| TEXAS INSTRUMENTS INCORPORATED
| Standard Linear and Logic Group
| IBIS Model of SN74LVC16646A
| 16-BIT REGISTERED TRANCEIVER AND REGISTER WITH 3-STATE OUTPUTS
| This file contains package information for the following:
|  TSSOP 56-pin (DGG) package as [Component] LVC16646A_DGG
|  TVSOP 56-pin (DGV) package as [Component] LVC16646A_DGV
|  SSOP 56-pin (DL) package as [Component] LVC16646A_DL
| This device can be powered at the following Vccs:
|  1.8 volt Vcc
|  2.5 volt Vcc
|  3.3 volt Vcc
| This file provides unique models under the [Model Selector] for each Vcc.
| For operation at a specific Vcc, select the appropriate model after each
| [Model Selector] keyword.
[IBIS Ver]   3.2
[Comment char]  |_char
[File Name]   sn74lvc16646a.ibs
[File Rev]   1.1 | c_die
[Date]   September 3, 2002
[Source]   Data created from TI-SPICE simulations at TI-SLL.
[Notes]   The following is an IBIS list for the LVC16646A.
   Please contact sllibis@ti.com with questions and
   comments concerning SLL IBIS models.
   This IBIS model is created from a BA (back annotated netlist
   - Power-clamp data has been deleted since there is no
   power-clamp diode in the device.
   - Due to the fact that the device is 5-V input/output
   tolerant, the pullup data has some non-monotonic warnings.
   - End point warning due to AC and DC mismatch.
[Disclaimer] Property of Texas Instruments Incorporated.  Unauthorized
   reproduction and/or distribution is strictly prohibited.
   This product is protected under copyright law.
   Created  2002, (C) Copyright  2002, Texas Instruments
   Incorporated, All Rights Reserved
   UNLESS THERE IS A SIGNED, WRITTEN AGREEMENT TO THE
   CONTRARY, TEXAS INSTRUMENTS (TI) IS PROVIDING THE IBIS
   MODELS  AND WITHOUT ANY WARRANTY, EXPRESSED OR
   IMPLIED.  TI assumes no liability for:
   1) the accuracy of the IBIS models provided to your
   company;
   2) the proper functioning of these IBIS Models in your
   design or for any resulting applications; or
   3) infringement of patents, copyrights or intellectual
   property rights resulting from your use of these IBIS
   models.
   TI provides IBIS Models as a service to our customers.
   You and your company shall not distribute, sell or give
   these models to anyone else without prior written
   permission from TI.
   TI reserves the right to make changes to our products or
   to discontinue any semiconductor product or service
   without notice, and advises our customers to obtain the
   latest version of relevant information to verify, before
   placing orders, that the information being relied on is
   current.
   Please be aware that your receipt and use of the IBIS
   information provided shall serve as acceptance of these
   terms and conditions.  If you do not accept these terms,
   you should return or destroy the IBIS models and any
   other accompanying information immediately.
| Component LVC16646A_DGG 56-pin TSSOP
[Component]   LVC16646A_DGG
[Manufacturer]   Texas Instruments, Inc.
[Package]
|   typ   min   max
R_pkg   4.500e-02   3.500e-02   6.200e-02
L_pkg   3.324e-09   2.403e-09   5.094e-09
C_pkg   5.640e-13   3.410e-13   9.140e-13
[Pin]   signal_name   model_name   R_pin   L_pin   C_pin
1   1DIR   LVC16646A_DIR   6.200e-02   5.094e-09   8.560e-13
2   1CLKAB   LVC16646A_CLK   6.100e-02   4.621e-09   9.020e-13
3   1SAB   LVC16646A_SEL   6.000e-02   4.316e-09   8.020e-13
4   GND   GND   5.900e-02   3.968e-09   6.980e-13
5   1A1   LVC16646A_IO   5.700e-02   3.716e-09   6.490e-13
6   1A2   LVC16646A_IO   4.200e-02   3.517e-09   6.520e-13
7   VCC   POWER   4.100e-02   3.160e-09   5.700e-13
8   1A3   LVC16646A_IO   3.900e-02   2.981e-09   4.820e-13
9   1A4   LVC16646A_IO   3.900e-02   2.809e-09   4.470e-13
10   1A5   LVC16646A_IO   3.800e-02   2.715e-09   4.090e-13
11   GND   GND   4.100e-02   2.675e-09   3.910e-13
12   1A6   LVC16646A_IO   3.900e-02   2.536e-09   3.660e-13
13   1A7   LVC16646A_IO   3.900e-02   2.457e-09   3.480e-13
14   1A8   LVC16646A_IO   3.800e-02   2.411e-09   3.530e-13
15   2A1   LVC16646A_IO   3.900e-02   2.456e-09   3.550e-13
16   2A2   LVC16646A_IO   3.900e-02   2.471e-09   3.490e-13
17   2A3   LVC16646A_IO   4.000e-02   2.580e-09   3.700e-13
18   GND   GND   3.800e-02   2.651e-09   3.890e-13
19   2A4   LVC16646A_IO   3.800e-02   2.739e-09   4.110e-13
20   2A5   LVC16646A_IO   3.900e-02   2.838e-09   4.490e-13
21   2A6   LVC16646A_IO   3.800e-02   2.988e-09   4.840e-13
22   VCC   POWER   3.800e-02   3.105e-09   5.640e-13
23   2A7   LVC16646A_IO   4.000e-02   3.427e-09   6.380e-13
24   2A8   LVC16646A_IO   5.600e-02   3.654e-09   6.410e-13
25   GND   GND   5.700e-02   3.932e-09   7.000e-13
26   2SAB   LVC16646A_SEL   5.800e-02   4.257e-09   8.060e-13
27   2CLKAB   LVC16646A_CLK   5.700e-02   4.580e-09   9.140e-13
28   2DIR   LVC16646A_DIR   5.900e-02   5.038e-09   8.610e-13
29   2NOE   LVC16646A_OE   6.000e-02   5.058e-09   8.580e-13
30   2CLKBA   LVC16646A_CLK   5.600e-02   4.543e-09   9.040e-13
31   2SBA   LVC16646A_SEL   5.700e-02   4.240e-09   8.030e-13
32   GND   GND   5.700e-02   3.929e-09   7.000e-13
33   2B8   LVC16646A_IO   5.600e-02   3.616e-09   6.370e-13
34   2B7   LVC16646A_IO   3.700e-02   3.368e-09   6.400e-13
35   VCC   POWER   3.600e-02   3.024e-09   5.630e-13
36   2B6   LVC16646A_IO   3.500e-02   2.876e-09   4.740e-13
37   2B5   LVC16646A_IO   3.500e-02   2.745e-09   4.440e-13
38   2B4   LVC16646A_IO   3.700e-02   2.683e-09   4.050e-13
39   GND   GND   3.800e-02   2.603e-09   3.820e-13
40   2B3   LVC16646A_IO   3.800e-02   2.510e-09   3.620e-13
41   2B2   LVC16646A_IO   3.600e-02   2.412e-09   3.410e-13
42   2B1   LVC16646A_IO   3.800e-02   2.416e-09   3.490e-13
43   1B8   LVC16646A_IO   3.700e-02   2.403e-09   3.490e-13
44   1B7   LVC16646A_IO   3.700e-02   2.429e-09   3.410e-13
45   1B6   LVC16646A_IO   3.600e-02   2.482e-09   3.580e-13
46   GND   GND   3.700e-02   2.615e-09   3.810e-13
47   1B5   LVC16646A_IO   3.500e-02   2.669e-09   4.020e-13
48   1B4   LVC16646A_IO   3.600e-02   2.763e-09   4.420e-13
49   1B3   LVC16646A_IO   3.600e-02   2.942e-09   4.780e-13
50   VCC   POWER   3.500e-02   3.053e-09   5.640e-13
51   1B2   LVC16646A_IO   3.600e-02   3.409e-09   6.410e-13
52   1B1   LVC16646A_IO   5.800e-02   3.698e-09   6.410e-13
53   GND   GND   5.900e-02   3.975e-09   6.970e-13
54   1SBA   LVC16646A_SEL   6.100e-02   4.327e-09   8.020e-13
55   1CLKBA   LVC16646A_CLK   6.100e-02   4.624e-09   9.050e-13
56   1NOE   LVC16646A_OE   6.000e-02   5.063e-09   8.580e-13
| Component LVC16646A_DGV 56-pin TVSOP
[Component]   LVC16646A_DGV
[Manufacturer]   Texas Instruments, Inc.
[Package]
|   typ   min   max
R_pkg   6.300e-02   5.000e-02   8.600e-02
L_pkg   2.945e-09   2.392e-09   3.938e-09
C_pkg   3.910e-13   2.710e-13   5.880e-13
[Pin]   signal_name   model_name   R_pin   L_pin   C_pin
1   1DIR   LVC16646A_DIR   6.800e-02   3.933e-09   5.880e-13
2   1CLKAB   LVC16646A_CLK   6.800e-02   3.569e-09   5.860e-13
3   1SAB   LVC16646A_SEL   7.600e-02   3.464e-09   5.150e-13
4   GND   GND   8.600e-02   3.451e-09   4.580e-13
5   1A1   LVC16646A_IO   8.200e-02   3.278e-09   4.260e-13
6   1A2   LVC16646A_IO   7.700e-02   3.143e-09   3.870e-13
7   VCC   POWER   6.900e-02   2.971e-09   4.010e-13
8   1A3   LVC16646A_IO   5.000e-02   2.787e-09   3.790e-13
9   1A4   LVC16646A_IO   5.100e-02   2.686e-09   3.200e-13
10   1A5   LVC16646A_IO   5.200e-02   2.607e-09   3.160e-13
11   GND   GND   5.300e-02   2.497e-09   2.970e-13
12   1A6   LVC16646A_IO   5.400e-02   2.438e-09   2.920e-13
13   1A7   LVC16646A_IO   5.500e-02   2.412e-09   2.860e-13
14   1A8   LVC16646A_IO   5.500e-02   2.400e-09   2.730e-13
15   2A1   LVC16646A_IO   5.500e-02   2.402e-09   2.730e-13
16   2A2   LVC16646A_IO   5.400e-02   2.398e-09   2.840e-13
17   2A3   LVC16646A_IO   5.400e-02   2.407e-09   2.890e-13
18   GND   GND   5.300e-02   2.448e-09   2.930e-13
19   2A4   LVC16646A_IO   5.200e-02   2.548e-09   3.110e-13
20   2A5   LVC16646A_IO   5.100e-02   2.623e-09   3.160e-13
21   2A6   LVC16646A_IO   5.000e-02   2.725e-09   3.700e-13
22   VCC   POWER   6.500e-02   2.903e-09   3.940e-13
23   2A7   LVC16646A_IO   7.300e-02   3.086e-09   3.870e-13
24   2A8   LVC16646A_IO   8.200e-02   3.272e-09   4.280e-13
25   GND   GND   8.200e-02   3.394e-09   4.570e-13
26   2SAB   LVC16646A_SEL   7.100e-02   3.374e-09   5.080e-13
27   2CLKAB   LVC16646A_CLK   6.900e-02   3.572e-09   5.810e-13
28   2DIR   LVC16646A_DIR   6.900e-02   3.937e-09   5.740e-13
29   2NOE   LVC16646A_OE   6.900e-02   3.923e-09   5.690e-13
30   2CLKBA   LVC16646A_CLK   6.800e-02   3.546e-09   5.740e-13
31   2SBA   LVC16646A_SEL   7.400e-02   3.422e-09   5.180e-13
32   GND   GND   8.100e-02   3.395e-09   4.680e-13
33   2B8   LVC16646A_IO   8.000e-02   3.255e-09   4.310e-13
34   2B7   LVC16646A_IO   7.100e-02   3.063e-09   3.860e-13
35   VCC   POWER   6.100e-02   2.878e-09   3.900e-13
36   2B6   LVC16646A_IO   5.000e-02   2.709e-09   3.640e-13
37   2B5   LVC16646A_IO   5.100e-02   2.607e-09   3.110e-13
38   2B4   LVC16646A_IO   5.100e-02   2.532e-09   3.060e-13
39   GND   GND   5.300e-02   2.440e-09   2.890e-13
40   2B3   LVC16646A_IO   5.300e-02   2.399e-09   2.860e-13
41   2B2   LVC16646A_IO   5.400e-02   2.392e-09   2.820e-13
42   2B1   LVC16646A_IO   5.500e-02   2.399e-09   2.710e-13
43   1B8   LVC16646A_IO   5.500e-02   2.395e-09   2.710e-13
44   1B7   LVC16646A_IO   5.500e-02   2.403e-09   2.830e-13
45   1B6   LVC16646A_IO   5.400e-02   2.421e-09   2.880e-13
46   GND   GND   5.300e-02   2.472e-09   2.920e-13
47   1B5   LVC16646A_IO   5.100e-02   2.569e-09   3.090e-13
48   1B4   LVC16646A_IO   5.100e-02   2.636e-09   3.130e-13
49   1B3   LVC16646A_IO   5.000e-02   2.739e-09   3.660e-13
50   VCC   POWER   6.500e-02   2.922e-09   3.900e-13
51   1B2   LVC16646A_IO   7.200e-02   3.076e-09   3.840e-13
52   1B1   LVC16646A_IO   8.100e-02   3.249e-09   4.300e-13
53   GND   GND   8.300e-02   3.400e-09   4.550e-13
54   1SBA   LVC16646A_SEL   7.300e-02   3.421e-09   5.060e-13
55   1CLKBA   LVC16646A_CLK   6.900e-02   3.579e-09   5.780e-13
56   1NOE   LVC16646A_OE   6.900e-02   3.938e-09   5.810e-13
| Component LVC16646A_DL 56-pin SSOP
[Component]   LVC16646A_DL
[Manufacturer]   Texas Instruments, Inc.
[Package]
|   typ   min   max
R_pkg   5.500e-02   4.800e-02   6.700e-02
L_pkg   6.539e-09   4.802e-09   9.746e-09
C_pkg   1.880e-13   7.600e-14   5.170e-13
[Pin]   signal_name   model_name   R_pin   L_pin   C_pin
1   1DIR   LVC16646A_DIR   6.400e-02   9.646e-09   5.130e-13
2   1CLKAB   LVC16646A_CLK   5.900e-02   8.723e-09   2.700e-13
3   1SAB   LVC16646A_SEL   5.900e-02   8.139e-09   2.230e-13
4   GND   GND   5.600e-02   7.554e-09   2.010e-13
5   1A1   LVC16646A_IO   5.400e-02   6.991e-09   1.950e-13
6   1A2   LVC16646A_IO   5.300e-02   6.659e-09   2.020e-13
7   VCC   POWER   5.500e-02   6.321e-09   2.070e-13
8   1A3   LVC16646A_IO   5.500e-02   5.942e-09   1.330e-13
9   1A4   LVC16646A_IO   5.700e-02   5.767e-09   1.320e-13
10   1A5   LVC16646A_IO   5.400e-02   5.459e-09   1.210e-13
11   GND   GND   5.100e-02   5.224e-09   1.400e-13
12   1A6   LVC16646A_IO   4.800e-02   5.088e-09   1.260e-13
13   1A7   LVC16646A_IO   5.000e-02   5.021e-09   9.600e-14
14   1A8   LVC16646A_IO   5.100e-02   4.802e-09   7.600e-14
15   2A1   LVC16646A_IO   5.100e-02   4.803e-09   7.600e-14
16   2A2   LVC16646A_IO   5.000e-02   5.021e-09   9.600e-14
17   2A3   LVC16646A_IO   4.800e-02   5.088e-09   1.260e-13
18   GND   GND   5.100e-02   5.224e-09   1.400e-13
19   2A4   LVC16646A_IO   5.400e-02   5.459e-09   1.210e-13
20   2A5   LVC16646A_IO   5.700e-02   5.768e-09   1.330e-13
21   2A6   LVC16646A_IO   5.500e-02   5.942e-09   1.330e-13
22   VCC   POWER   5.500e-02   6.320e-09   2.060e-13
23   2A7   LVC16646A_IO   5.300e-02   6.659e-09   2.030e-13
24   2A8   LVC16646A_IO   5.400e-02   6.991e-09   1.960e-13
25   GND   GND   5.600e-02   7.554e-09   2.010e-13
26   2SAB   LVC16646A_SEL   5.900e-02   8.139e-09   2.230e-13
27   2CLKAB   LVC16646A_CLK   5.900e-02   8.727e-09   2.700e-13
28   2DIR   LVC16646A_DIR   6.700e-02   9.746e-09   5.170e-13
29   2NOE   LVC16646A_OE   6.300e-02   9.630e-09   5.110e-13
30   2CLKBA   LVC16646A_CLK   6.000e-02   8.751e-09   2.710e-13
31   2SBA   LVC16646A_SEL   6.000e-02   8.184e-09   2.250e-13
32   GND   GND   5.600e-02   7.543e-09   2.000e-13
33   2B8   LVC16646A_IO   5.400e-02   7.005e-09   1.960e-13
34   2B7   LVC16646A_IO   5.600e-02   6.714e-09   2.040e-13
35   VCC   POWER   5.800e-02   6.384e-09   2.080e-13
36   2B6   LVC16646A_IO   5.700e-02   5.976e-09   1.340e-13
37   2B5   LVC16646A_IO   5.700e-02   5.743e-09   1.300e-13
38   2B4   LVC16646A_IO   5.400e-02   5.468e-09   1.190e-13
39   GND   GND   5.500e-02   5.328e-09   1.420e-13
40   2B3   LVC16646A_IO   5.200e-02   5.189e-09   1.290e-13
41   2B2   LVC16646A_IO   5.200e-02   5.053e-09   9.600e-14
42   2B1   LVC16646A_IO   5.100e-02   4.825e-09   7.600e-14
43   1B8   LVC16646A_IO   5.400e-02   4.896e-09   7.800e-14
44   1B7   LVC16646A_IO   5.200e-02   5.093e-09   9.700e-14
45   1B6   LVC16646A_IO   5.100e-02   5.179e-09   1.280e-13
46   GND   GND   5.400e-02   5.314e-09   1.420e-13
47   1B5   LVC16646A_IO   5.500e-02   5.511e-09   1.210e-13
48   1B4   LVC16646A_IO   5.700e-02   5.771e-09   1.310e-13
49   1B3   LVC16646A_IO   5.600e-02   5.957e-09   1.330e-13
50   VCC   POWER   5.500e-02   6.320e-09   2.060e-13
51   1B2   LVC16646A_IO   5.200e-02   6.621e-09   2.000e-13
52   1B1   LVC16646A_IO   5.300e-02   6.973e-09   1.950e-13
53   GND   GND   5.700e-02   7.571e-09   2.020e-13
54   1SBA   LVC16646A_SEL   5.700e-02   8.097e-09   2.220e-13
55   1CLKBA   LVC16646A_CLK   5.900e-02   8.723e-09   2.710e-13
56   1NOE   LVC16646A_OE   6.100e-02   9.560e-09   5.090e-13
| Model LVC16646A_SEL
[Model Selector]   LVC16646A_SEL
LVC16646A_SEL_18   1.8 volt Vcc
LVC16646A_SEL_25   2.5 volt Vcc
LVC16646A_SEL_33   3.3 volt Vcc
| Model LVC16646A_DIR
[Model Selector]   LVC16646A_DIR
LVC16646A_DIR_18   1.8 volt Vcc
LVC16646A_DIR_25   2.5 volt Vcc
LVC16646A_DIR_33   3.3 volt Vcc
| Model LVC16646A_CLK
[Model Selector]   LVC16646A_CLK
LVC16646A_CLK_18   1.8 volt Vcc
LVC16646A_CLK_25   2.5 volt Vcc
LVC16646A_CLK_33   3.3 volt Vcc
| Model LVC16646A_OE
[Model Selector]   LVC16646A_OE
LVC16646A_OE_18   1.8 volt Vcc
LVC16646A_OE_25   2.5 volt Vcc
LVC16646A_OE_33   3.3 volt Vcc
| Model LVC16646A_IO
[Model Selector]   LVC16646A_IO
LVC16646A_IO_18   1.8 volt Vcc
LVC16646A_IO_25   2.5 volt Vcc
LVC16646A_IO_33   3.3 volt Vcc
| Models and submodels in the file (15): LVC16646A_SEL_18 (Input), LVC16646A_SEL_25 (Input), LVC16646A_SEL_33 (Input), LVC16646A_DIR_18 (Input), LVC16646A_DIR_25 (Input), LVC16646A_DIR_33 (Input), LVC16646A_CLK_18 (Input), LVC16646A_CLK_25 (Input), LVC16646A_CLK_33 (Input), LVC16646A_OE_18 (Input), LVC16646A_OE_25 (Input), LVC16646A_OE_33 (Input), LVC16646A_IO_18 (I/O), LVC16646A_IO_25 (I/O), LVC16646A_IO_33 (I/O)
